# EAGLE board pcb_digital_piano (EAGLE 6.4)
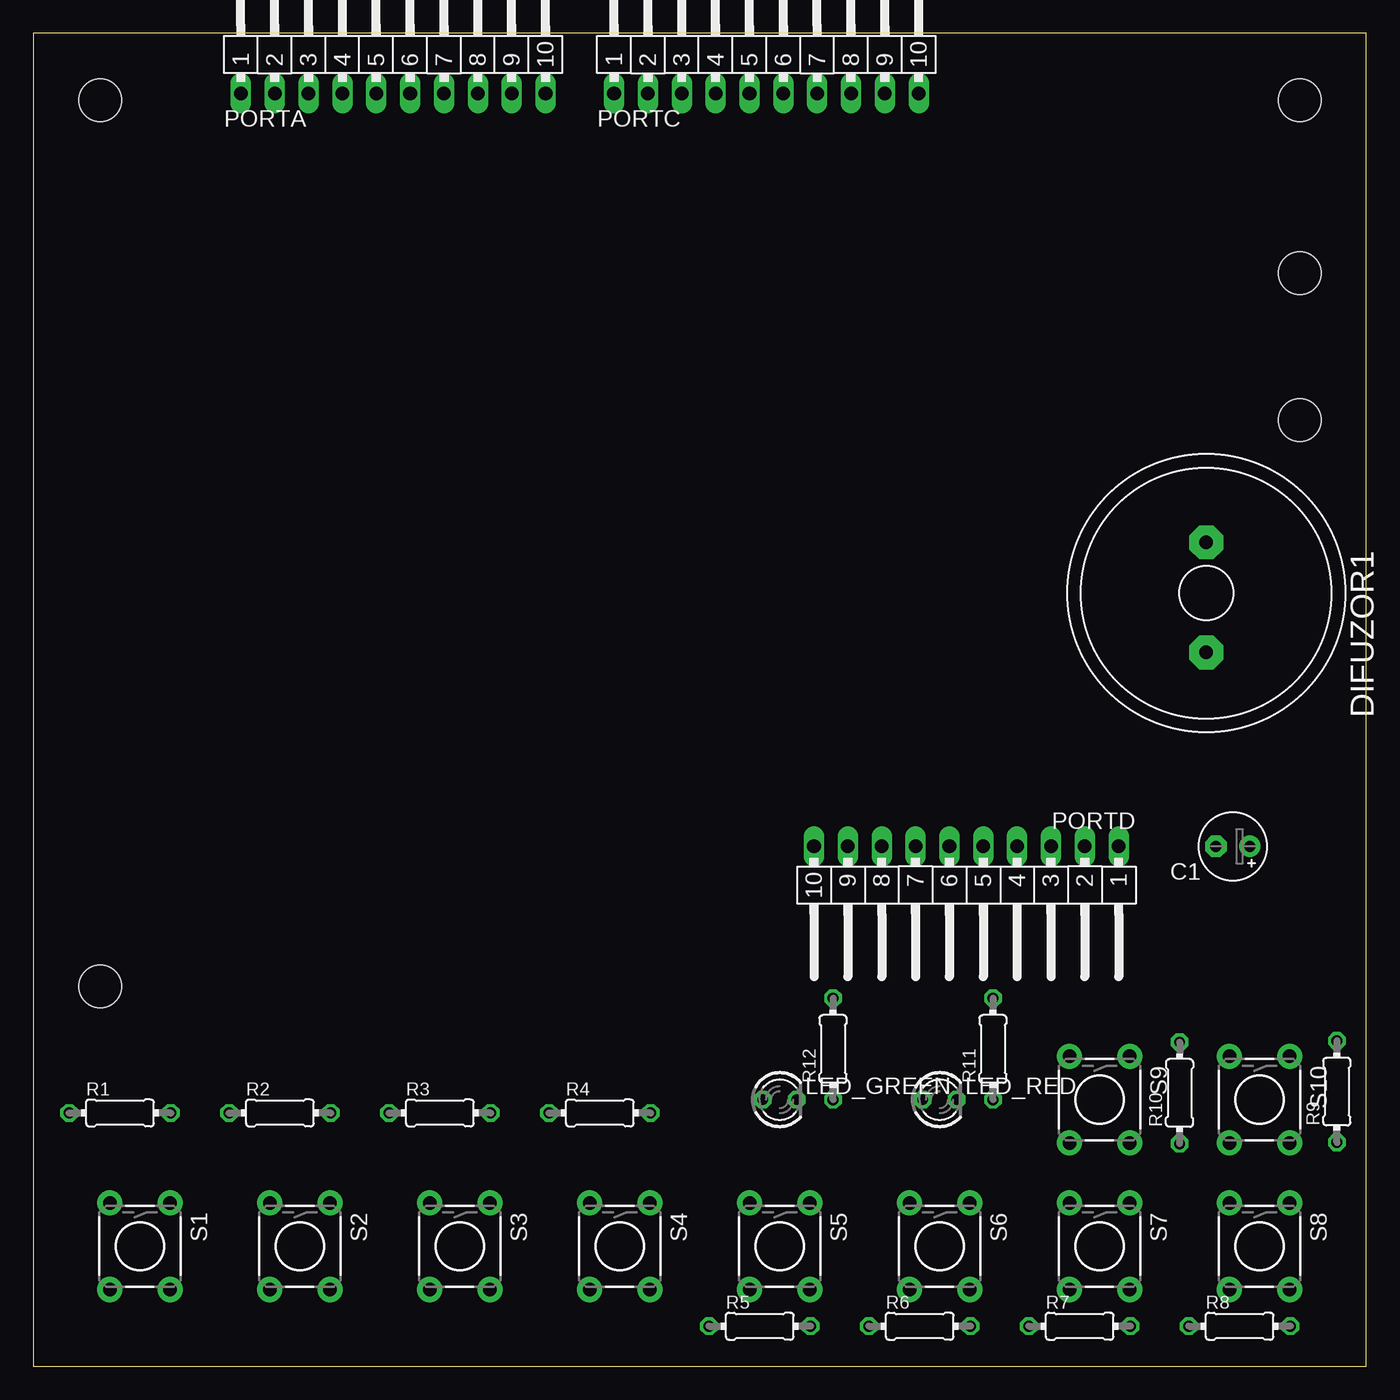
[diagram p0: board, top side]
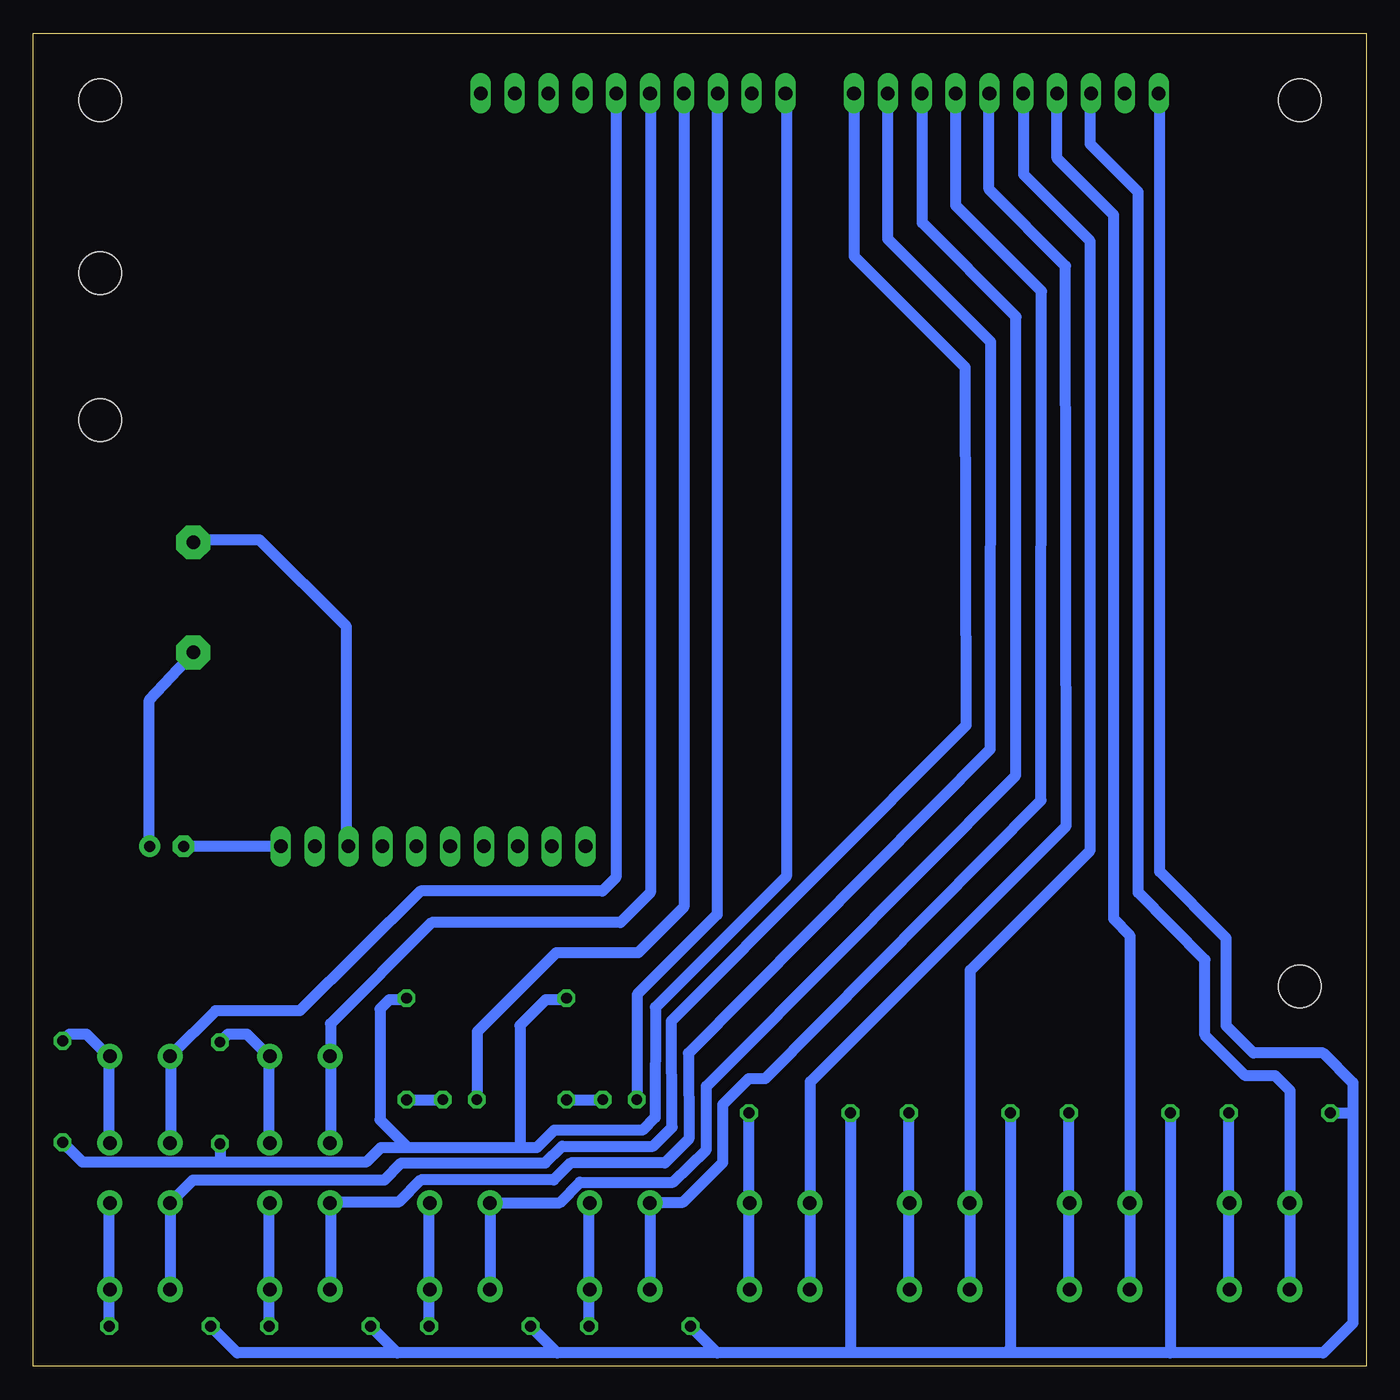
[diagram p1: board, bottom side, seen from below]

Size 100 x 100 mm. Coordinates in mm from the lower left corner, seen from the top.
Outline: 0,0 100,0 100,100 0,100 0,0
Copper layers (1*16): Top 0.8mm / dielectric 1.5mm / Bottom 0.8mm
Design rules "default": minimum track width 14mil, minimum drill 24mil, track to track 12mil, track to pad 12mil, pad to pad 12mil, via to via 12mil, smd to smd 8mil, copper to edge 40mil, drill to drill 8mil, minimum pad ring 10mil, minimum via ring 8mil, stop-mask expansion 4mil, vias tented up to drill 0mil, thermal gap 10mil
Holes 3.2 mm at 5,95 5,28.5 95,71 95,95 95,82

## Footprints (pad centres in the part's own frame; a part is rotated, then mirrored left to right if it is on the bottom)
E2,5-5 = drill 0.813 pad 1.6: + -1.27,0 | drill 0.813 pad 1.6 octagon: - 1.27,0
AL201P = drill 1.016 pad 2.54 octagon: 1 -3.81,0; 2 4.445,0
LED3MM = drill 0.813 octagon: A -1.27,0; K 1.27,0
MA10-1W = drill 1.016 long: 1 -11.43,0; 2 -8.89,0; 3 -6.35,0; 4 -3.81,0; 5 -1.27,0; 6 1.27,0; 7 3.81,0; 8 6.35,0; 9 8.89,0; 10 11.43,0
0204/7 = drill 0.813 octagon: 1 -3.81,0; 2 3.81,0
TACTILE-PTH = drill 1.016 pad 1.88: 1 -3.251,2.261; 2 3.251,2.261; 3 -3.251,-2.261; 4 3.251,-2.261

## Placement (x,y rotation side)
C1  100uF  [E2,5-5]  90,39 180 top
DIFUZOR1  AL201P  [AL201P]  88,58 270 top
LED_GREEN  TLLR4400  [LED3MM]  56,20 0 top
LED_RED  TLLR4400  [LED3MM]  68,20 0 top
PORTA  [MA10-1W]  27,95.5 0 top
PORTC  [MA10-1W]  55,95.5 0 top
PORTD  [MA10-1W]  70,39 180 top
R1  100  [0204/7]  6.5,19 0 top
R2  100  [0204/7]  18.5,19 0 top
R3  100  [0204/7]  30.5,19 0 top
R4  100  [0204/7]  42.5,19 0 top
R5  100  [0204/7]  54.5,3 0 top
R6  100  [0204/7]  66.5,3 0 top
R7  100  [0204/7]  78.5,3 0 top
R8  100  [0204/7]  90.5,3 0 top
R9  100  [0204/7]  97.8,20.6 90 top
R10  100  [0204/7]  86,20.5 90 top
R11  1k  [0204/7]  72,23.8 90 top
R12  1k  [0204/7]  60,23.8 90 top
S1  [TACTILE-PTH]  8,9 270 top
S2  [TACTILE-PTH]  20,9 270 top
S3  [TACTILE-PTH]  32,9 270 top
S4  [TACTILE-PTH]  44,9 270 top
S5  [TACTILE-PTH]  56,9 270 top
S6  [TACTILE-PTH]  68,9 270 top
S7  [TACTILE-PTH]  80,9 270 top
S8  [TACTILE-PTH]  92,9 270 top
S9  [TACTILE-PTH]  80,20 270 top
S10  [TACTILE-PTH]  92,20 270 top

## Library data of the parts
C1 R1-R12 = resistor
DIFUZOR1 = buzzer; OC_FARNELL: unknown; OC_NEWARK: unknown
LED_GREEN LED_RED = led; MF: VISHAY SEMICONDUCTOR; OC_FARNELL: 1612437
PORTA PORTC PORTD = con-lstb; OC_FARNELL: unknown; OC_NEWARK: unknown
S1-S10 = SparkFun

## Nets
+5V(A)1: PORTC.2
+5V(C): PORTA.2
+5V(D): PORTD.2
N$13: S3.2
N$17: S6.2
N$18: S9.3
N$19: S10.3
N$20: S8.2
N$21: S1.3
N$22: S3.3
N$23: S5.3
N$24: S7.3
PA8: PORTC.10
PA9: PORTC.9
PA10: PORTC.8
PD0: PORTD.10
PD1: PORTD.9
PD2: PORTD.8
PD3: PORTD.7
PD4: PORTD.6
PD6: PORTD.4
PD7: PORTD.3

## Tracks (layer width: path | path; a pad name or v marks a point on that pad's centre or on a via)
S$2
  Bottom 0.813: 81.5,39 89,39
S$3
  Bottom 0.813: 1,19 1,21.26 3.24,23.5 8.45,23.5 10.5,25.55 10.5,32.1 15.5,37.12 15.5,95.5 | 1,19 1,3.24 3.24,1 14.7,1 | 14.7,1 48.7,1 | 48.7,1 60.7,1 | 60.7,1 72.7,1 | 72.7,1 84.7,1 86.7,3 | 2.7,19 1,19 | 74.7,3 72.7,1 | 62.7,3 60.7,1 | 50.7,3 48.7,1 | 14.7,19 14.7,1
S$4
  Bottom 0.813: 10.3,5.7 10.3,19
S$5
  Bottom 0.813: 5.7,5.7 5.7,20.67 6.83,21.8 9.07,21.8 12.1,24.83 12.1,30.5 17.1,35.54 17.1,88.09 20.7,91.69 20.7,95.5
S$6
  Bottom 0.813: 22.3,5.7 22.3,19.1
S$7
  Bottom 0.813: 34.3,5.7 34.3,19.1
S$8
  Bottom 0.813: 46.3,5.7 46.3,19.1
S$9
  Bottom 0.813: 41.7,5.7 41.7,21.34 22.5,40.54 22.55,82.55 28.3,88.3 28.3,95.5
S$10
  Bottom 0.813: 17.7,5.74 17.7,32.28 18.95,33.56 18.95,86.36 23.2,90.61 23.2,95.5
S$11
  Bottom 0.813: 29.7,5.7 29.7,29.7 20.7,38.7 20.7,84.4 25.7,89.4 25.7,95.5
S$12
  Bottom 0.813: 53.7,5.7 53.7,12.29 51.24,12.29 48.26,15.29 48.26,19.64 46.31,21.59 45.09,21.59 24.4,42.45 24.36,80.64 30.8,87.08 30.8,95.5
S$13
  Bottom 0.813: 58.3,3.2 58.3,12.6
S$14
  Bottom 0.813: 65.7,5.7 65.7,12.27 60.5,12.27 59,13.8 52,13.8 49.5,16.23 49.5,21 47.62,22.86 26.3,44.33 26.27,78.74 33.3,85.78 33.3,95.5
S$15
  Bottom 0.813: 70.3,3 70.3,12.4
S$16
  Bottom 0.813: 43.5,95.5 43.5,36.73 53.32,26.92 53.34,18.66 54.3,17.7 60.93,17.7 62.23,16.4 73.94,16.4 75.03,15.3 96.3,15.3 97.8,16.8
S$17
  Bottom 0.813: 82.3,3 82.3,12.4
S$18
  Bottom 0.813: 89.7,5.7 89.7,12.29 88.02,13.97 73.66,13.97 72.39,15.24 61.59,15.24 60.33,16.51 53.5,16.51 52.08,17.94 52.12,25.89 30,48.1 30.07,74.93 38.4,83.25 38.4,95.5
S$19
  Bottom 0.813: 94.3,3 94.3,12.4
S$20
  Bottom 0.813: 26.7,19 26.7,1.4
S$21
  Bottom 0.813: 38.7,19 38.7,1.3
S$22
  Bottom 0.813: 48.7,95.5 48.7,33.88 54.7,27.88 54.7,20
S$23
  Bottom 0.813: 35.9,95.5 35.9,84.56 28.17,76.83 28.2,46.3 50.86,23.47 50.81,17.05 52.61,15.24 59.69,15.24 60.96,13.97 70.94,13.97 72.61,12.3 77.7,12.3 77.7,5.7
S$24
  Bottom 0.813: 60,20 57,20
S$25
  Bottom 0.813: 72,20 69,20
S$26
  Bottom 0.813: 60,27.5 61.56,27.5 63.5,25.56 63.5,16.5
S$27
  Bottom 0.813: 72,27.5 73.29,27.5 74,26.79 74,18.5 72,16.5
S$28
  Bottom 0.813: 86,16.7 86,15.5
S$29
  Bottom 0.813: 94.3,16.7 94.3,23.2 96,24.9 97.3,24.9 97.8,24.4
S$30
  Bottom 0.813: 82.3,16.7 82.3,23.24 83.96,24.9 85.4,24.9 86,24.3
S$31
  Bottom 0.813: 51.2,95.5 51.2,34.44 54.62,31.02 60.78,31.02 66.7,25.1 66.7,20
S$32
  Bottom 0.813: 53.7,95.5 53.7,35.54 55.95,33.28 70.11,33.28 77.7,25.69 77.7,16.6
S$33
  Bottom 0.813: 56.3,95.5 56.3,36.66 57.31,35.66 70.95,35.66 80.01,26.67 86.33,26.67 89.7,23.3 89.7,16.6
S$34
  Bottom 0.813: 91.3,39 91.3,50 88,53.5
S$35
  Bottom 0.813: 76.5,39 76.5,55.48 83.02,62 88,62

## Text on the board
_tsilk: 1 | 2 | 3 | 4 | 5 | 6 | 7 | 8 | 9 | 10 | 1 | 2 | 3 | 4 | 5 | 6 | 7 | 8 | 9 | 10 | R1 | PORTC | 1k | PORTA | TLLR4400 | TLLR4400 | R2 | 1k | LED1 | LED2 | S1 | S2 | S3 | R3 | R5 | 100 | 100 | 100 | R4 | PORTD | 1 | 2 | C1 | 3 | 100uF | 4 | 5 | SP1 | 6 | AL201P | 7 | 8 | 9 | 10 | S4 | S5 | S6 | S7 | S8 | S9 | S10 | S11 | R6 | R7 | R8 | R9 | R10 | R11 | R12 | R13 | 1k | 1k | 100 | 100 | 100 | 100 | 100 | 100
